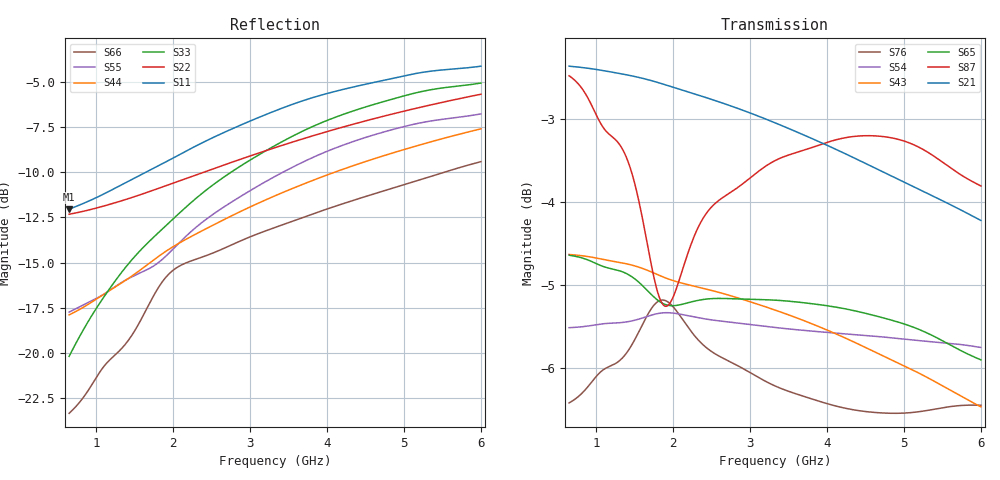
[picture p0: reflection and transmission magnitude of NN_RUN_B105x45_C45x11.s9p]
! IGNION VIRTUAL ANTENNA LIBRARY
! NN_RUN_B105x45_C45x11
! Virtual Antenna™ RUN mXTEND™: NN02-224 12.0 mm x 3.0 mm x 2.4 mm
! https://ignion.io/product/run-mxtend/
! Board: 105 mm x 45 mm
! Clearance Area: 45 mm x 11 mm
! Feeding line: L-shape; 11mm x 2mm and 5mm x 2mm
! Applications: Fleet management, IoT
! Frequency range 0.65GHz to 6GHz, step 10MHz
! Number of ports 9
! This product and its use is protected by at least one or more of the following patents and patent
! applications US 8,203,492 B2; US 8,237,615 B2; PCT/EP2013/064692; WO 2014/012842 A1; US 2019/190122 A1;
! US 62/072,671; and other domestic and international patents pending. Additional information about
! patents related to this product is available at https://ignion.io/files/Patent-list-NN.pdf, all
! rights reserved. Copyright, Ignion 2021.
! Need more help? Your platform is much different than these examples in the manual? Use our
! Fast Track service (https://ignion.io/fast-track/), for free, and get a personalized antenna design in
! just 24 hours.
! Touchstone port 1 = "Series Port"
! Touchstone port 2 = "Shunt Port"
! Touchstone port 3 = "Series Port"
! Touchstone port 4 = "Shunt Port"
! Touchstone port 5 = "Series Port"
! Touchstone port 6 = "Shunt Port"
! Touchstone port 7 = "Series Port"
! Touchstone port 8 = "Shunt Port"
! Touchstone port 9 = "Series Port"
! IE3D S-Parameters Output Version 2.0
# GHZ S MA R 50
! Nport = 9
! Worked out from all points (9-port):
!   536 points, 650 MHz to 6 GHz, reference 50 ohm
!   strongest paths, dB at 650 MHz, 1.99 GHz, 3.33 GHz, 4.67 GHz, 6 GHz:
!     S21: -2.4, -2.6, -3.0, -3.6, -4.2
!     S87: -2.5, -5.2, -3.5, -3.2, -3.8
!     S65: -4.6, -5.3, -5.2, -5.4, -5.9
!     S43: -4.6, -4.9, -5.3, -5.8, -6.5
!     S54: -5.5, -5.3, -5.5, -5.6, -5.8
!     S76: -6.4, -5.3, -6.2, -6.5, -6.5
!   lowest |S11| = -12.0 dB at 650 MHz (marker M1), VSWR 1.67, Z = 31.1 + j7.76 ohm
!   |S11| at or under -10 dB: start of sweep to 1.644 GHz
